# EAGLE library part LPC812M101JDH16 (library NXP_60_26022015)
32-bit ARM Cortex-M0+ microcontroller The LPC81xM are an ARM Cortex-M0+ based, low-cost 32-bit MCU family operating at CPU frequencies of up to 30 MHz. The LPC81xM support up to 16 kB of flash memory and 4 kB of SRAM. The peripheral complement of the LPC81xM includes a CRC engine, one I 2 C-bus interface, up to three USARTs, up to two SPI interfaces, one multi-rate timer, self wake-up timer, and state-configurable timer, one comparator, function-configurable I/O ports through a switch matrix, an input pattern match engine, and up to 18 general-purpose I/O pins. AAL Eindhoven MK
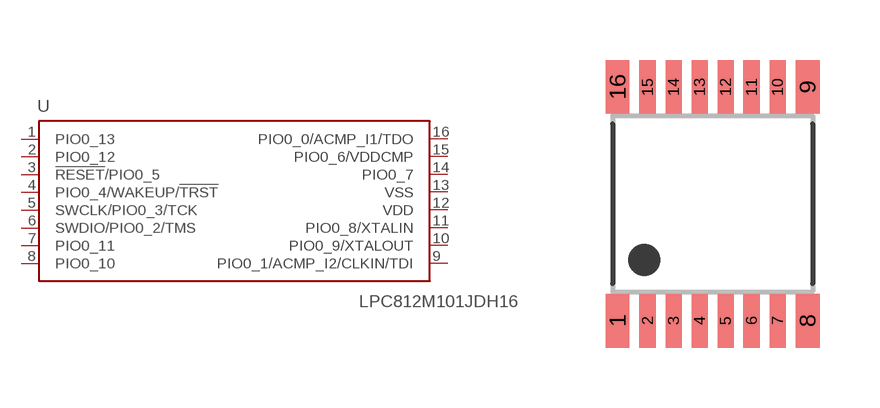
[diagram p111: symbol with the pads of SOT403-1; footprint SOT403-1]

Designator prefix U

## LPC812M101JDH16 (COMP: 1; FLASH: 16k; GPIO: 14; I2C: 1; SPI: 2; SRAM: 4k; USART: 3)  [SOT403-1]
1  PIO0_13
2  PIO0_12
3  !RESET!/PIO0_5
4  PIO0_4/WAKEUP/!TRST!
5  SWCLK/PIO0_3/TCK
6  SWDIO/PIO0_2/TMS
7  PIO0_11
8  PIO0_10
9  PIO0_1/ACMP_I2/CLKIN/TDI
10  PIO0_9/XTALOUT
11  PIO0_8/XTALIN
12  VDD  pwr
13  VSS  pwr
14  PIO0_7
15  PIO0_6/VDDCMP
16  PIO0_0/ACMP_I1/TDO

## Footprint SOT403-1 (pad centres in mm)
SOT403-1 TSSOP16: plastic thin shrink small outline package; 16 leads; body width 4.4 mm JEDEC: MO-153 IEC: ---
smd 0.6 x 1.35: 1 -2.375,-2.925; 8 2.375,-2.925; 9 2.375,2.925; 16 -2.375,2.925
smd 0.4 x 1.35: 2 -1.625,-2.925; 3 -0.975,-2.925; 4 -0.325,-2.925; 5 0.325,-2.925; 6 0.975,-2.925; 7 1.625,-2.925; 10 1.625,2.925; 11 0.975,2.925; 12 0.325,2.925; 13 -0.325,2.925; 14 -0.975,2.925; 15 -1.625,2.925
